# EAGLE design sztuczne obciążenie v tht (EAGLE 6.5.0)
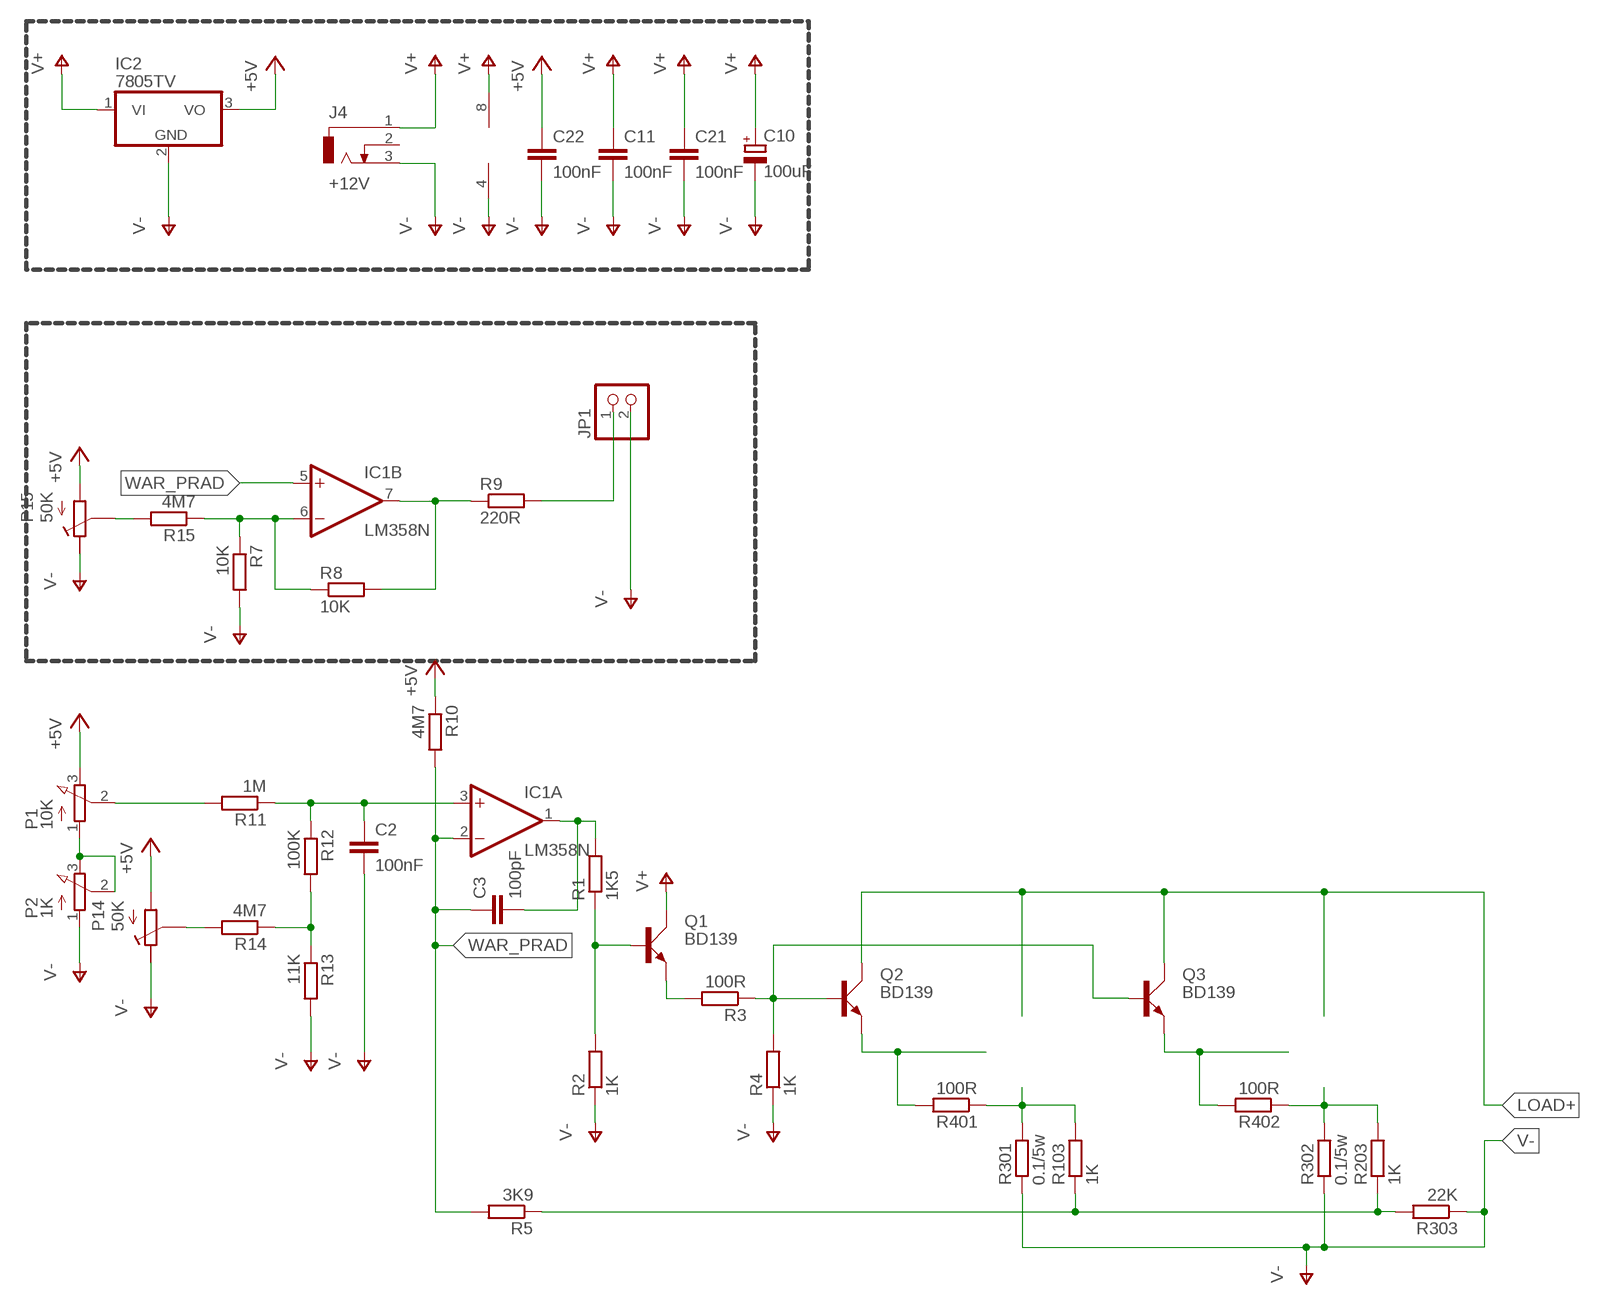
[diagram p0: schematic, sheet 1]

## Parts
C2  100nF  C-EU025-025X050  [C025-025X050]
C3  100pF  C-EU025-025X050  [C025-025X050]
C10  100uF  CPOL-EUE5-10.5  [E5-10,5]
C11  100nF  C-EU025-025X050  [C025-025X050]
C21  100nF  C-EU025-025X050  [C025-025X050]
C22  100nF  C-EU025-025X050  [C025-025X050]
IC1  LM358N  [DIL08]
IC2  7805TV  [TO220V]
J4  +12V  DCJ0202  [DCJ0202]
JP1  PINHD-1X2  [1X02]
P1  10K  3RP/1610N  [3RP/1610N]
P2  1K  3RP/1610N  [3RP/1610N]
P14  50K  POTENCJOMETR_RM-065  [RM065]
P15  50K  POTENCJOMETR_RM-065  [RM065]
Q1  BD139  [TO126AV]
Q2  BD139  [TO126AV]
Q3  BD139  [TO126AV]
R1  1K5  R-EU_0207/7  [0207/7]
R2  1K  R-EU_0207/7  [0207/7]
R3  100R  R-EU_0207/7  [0207/7]
R4  1K  R-EU_0207/7  [0207/7]
R5  3K9  R-EU_0207/7  [0207/7]
R7  10K  R-EU_0207/7  [0207/7]
R8  10K  R-EU_0207/7  [0207/7]
R9  220R  R-EU_0207/7  [0207/7]
R10  4M7  R-EU_0207/7  [0207/7]
R11  1M  R-EU_0207/7  [0207/7]
R12  100K  R-EU_0207/7  [0207/7]
R13  11K  R-EU_0207/7  [0207/7]
R14  4M7  R-EU_0207/7  [0207/7]
R15  4M7  R-EU_0207/7  [0207/7]
R103  1K  R-EU_0207/7  [0207/7]
R203  1K  R-EU_0207/7  [0207/7]
R301  0.1/5w  R-EU_0922/22  [0922/22]
R302  0.1/5w  R-EU_0922/22  [0922/22]
R303  22K  R-EU_0207/7  [0207/7]
R401  100R  R-EU_0207/7  [0207/7]
R402  100R  R-EU_0207/7  [0207/7]

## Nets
+5V: C22.1 IC2.3(VO) P1.3(E) P14.P$3(A) P15.P$3(A) R10.1
LOAD+: Q2.C Q3.C
N$2: R203.2 R302.2 R402.1
N$3: Q2.B Q3.B R3.1 R4.2
N$4: Q2.E R401.2
N$5: Q1.B R1.1 R2.2
N$7: JP1.1 R9.2
N$8: C3.2 IC1.1(A:OUT) R1.2
N$9: P1.2(S) R11.2
N$10: C2.1 IC1.3(A:+IN) R11.1 R12.1
N$11: R12.2 R13.1 R14.1
N$12: Q1.E R3.2
N$13: Q3.E R402.2
N$14: R5.1 R103.1 R203.1 R303.2
N$15: P14.P$1(S) R14.2
N$16: IC1.6(B:-IN) R7.1 R8.1 R15.1
N$17: P15.P$1(S) R15.2
N$18: R103.2 R301.2 R401.1
N$19: IC1.7(B:OUT) R8.2 R9.1
N$26: P1.1(A) P2.2(S) P2.3(E)
V+: C10.+ C11.1 C21.1 IC1.8(P:V+) IC2.1(VI) J4.1 Q1.C
V-: C2.2 C10.- C11.2 C21.2 C22.2 IC1.4(P:V-) IC2.2(GND) J4.3 JP1.2 P2.1(A) P14.P$2(E) P15.P$2(E) R2.1 R4.1 R7.2 R13.2 R301.1 R302.1 R303.1
WAR_PRAD: C3.1 IC1.2(A:-IN) IC1.5(B:+IN) R5.2 R10.2
Unconnected: J4.2

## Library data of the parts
C2 C3 C11 C21 C22 = rcl:C-EU: CAPACITOR, European symbol
C10 = rcl:CPOL-EU: POLARIZED CAPACITOR, European symbol
IC1 = linear:LM358: OP AMP also LM158; LM258; LM2904 Source: http://cache.national.com/ds/LM/LM158.pdf
IC2 = linear:78*: Positive VOLTAGE REGULATOR Source: http://cache.national.com/ds/LM/LM78L05.pdf http://www.fairchildsemi.com/ds/LM/LM7805.pdf
J4 = con-jack:DCJ0202: DC POWER JACK Source: DCJ0202.pdf; OC_FARNELL: unknown; OC_NEWARK: unknown
JP1 = pinhead:PINHD-1X2: PIN HEADER
P1 P2 = pot:3RP/1610N: 16mm Potentiometer one level Source: http://www.alphapotentiometers.net/html/16mm_pot_2.html
P14 P15 = POT_RM065:POTENCJOMETR_RM-065
Q1-Q3 = transistor-power:BD139: NPN TRANSISTOR
R1-R5 R7-R15 R103 R203 R301-R303 R401 R402 = resistor:R-EU_: RESISTOR, European symbol

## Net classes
1 pradowa: width 1.524 mm, clearance 0.508 mm
2 srednia: width 0.635 mm

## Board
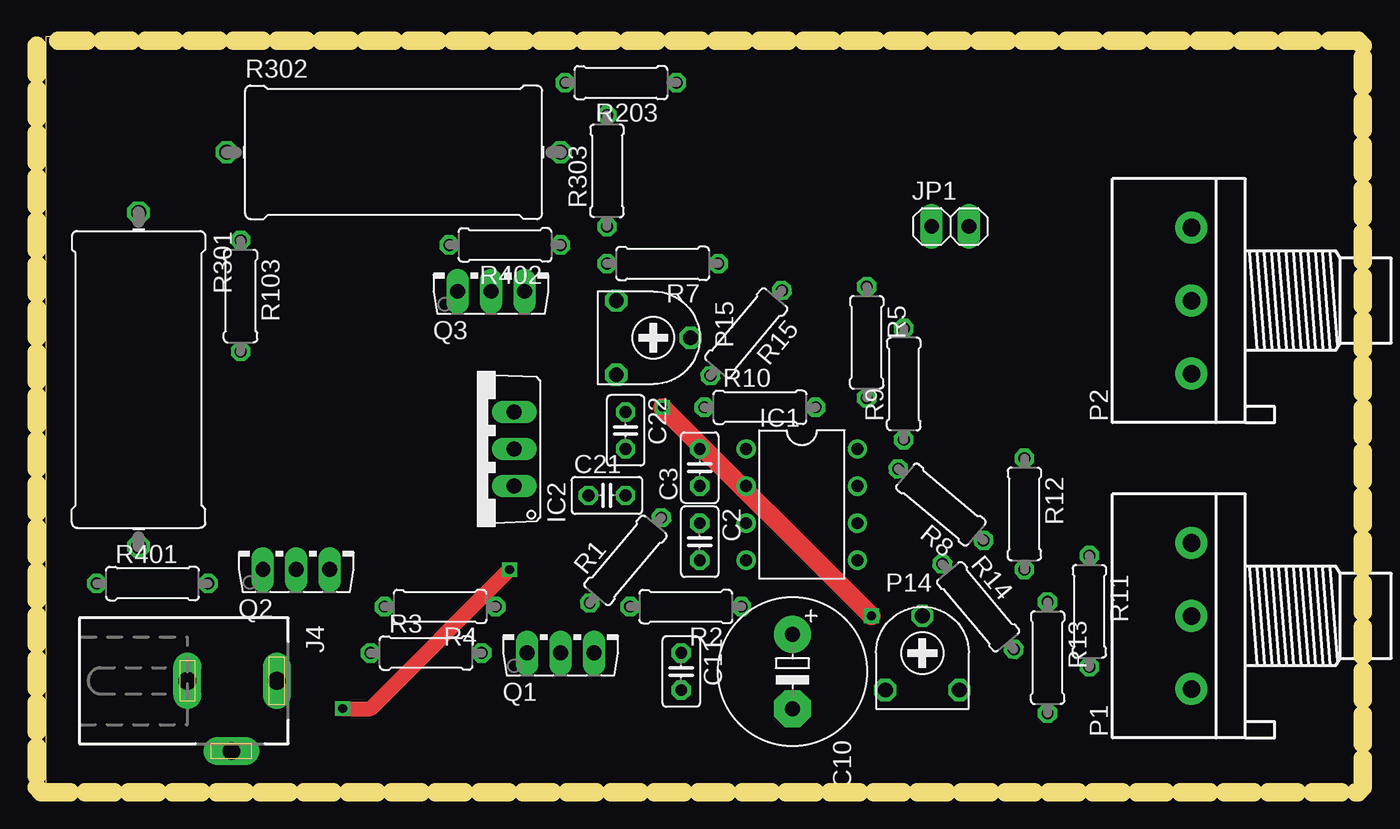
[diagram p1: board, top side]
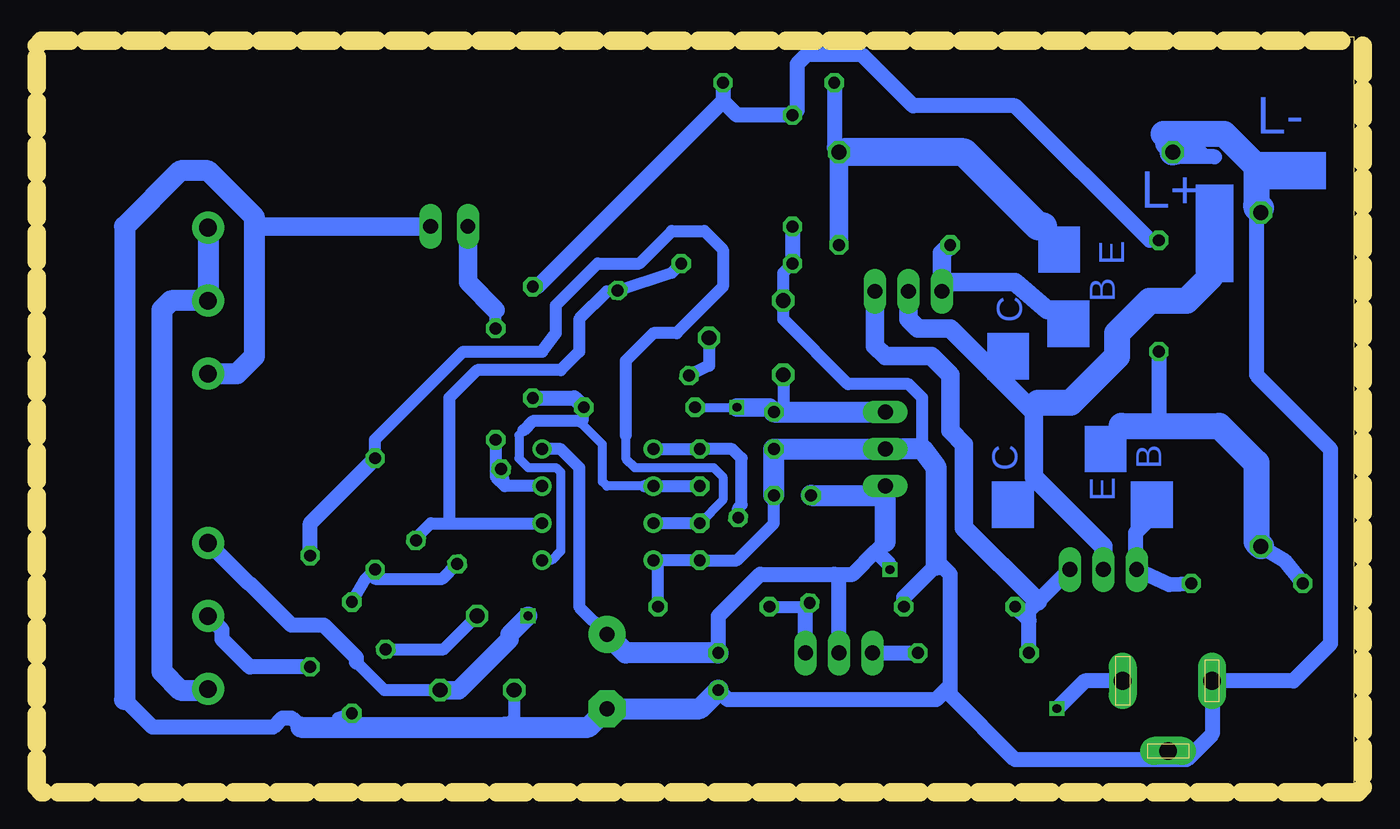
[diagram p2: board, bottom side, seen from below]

Size 90.81 x 51.74 mm. Coordinates in mm from the lower left corner, seen from the top.
Outline: 0.64,51.44 0.64,51.74 90.79,51.74 90.79,0.32 0.64,0 0.64,51.44
Outline: 0,51.12 0,0.32 0.32,0 90.49,0 90.81,0.32 90.81,51.12 90.49,51.44 0.64,51.44
Copper layers (1*16): Top 0.035mm / dielectric 1.5mm / Bottom 0.035mm
Design rules "default": minimum track width 10mil, minimum drill 24mil, track to track 8mil, track to pad 8mil, pad to pad 8mil, via to via 8mil, smd to smd 8mil, copper to edge 40mil, drill to drill 8mil, minimum pad ring 10mil, minimum via ring 8mil, stop-mask expansion 4mil, vias tented up to drill 0mil, thermal gap 10mil

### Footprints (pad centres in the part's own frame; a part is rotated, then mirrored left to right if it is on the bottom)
C025-025X050 = drill 0.813 octagon: 1 -1.27,0; 2 1.27,0
E5-10,5 = drill 1.016 pad 2.54: + -2.54,0 | drill 1.016 pad 2.54 octagon: - 2.54,0
DIL08 = drill 0.813 pad 1.27: 1 -3.81,-3.81; 2 -1.27,-3.81; 3 1.27,-3.81; 4 3.81,-3.81; 5 3.81,3.81; 6 1.27,3.81; 7 -1.27,3.81; 8 -3.81,3.81
TO220V = drill 1.016 long: 1 -2.54,-2.54; 2 0,-2.54; 3 2.54,-2.54
DCJ0202 = drill 1.2 pad 1.93 long: 1 0,3.105; 2 4.8,0; 3 0,-3.015
1X02 = drill 1.016 long: 1 -1.27,0; 2 1.27,0
3RP/1610N = drill 1.2 pad 2.184: 1 -5,0; 2 0,0; 3 5,0
RM065 = drill 1.016 octagon: P$1 0,2.54; P$2 -2.54,-2.54; P$3 2.54,-2.54
TO126AV = drill 1.016 long: B 2.286,-1.27; C 0,-1.27; E -2.286,-1.27
0207/7 = drill 0.813 octagon: 1 -3.81,0; 2 3.81,0
0922/22 = drill 1.016 octagon: 1 -11.43,0; 2 11.43,0

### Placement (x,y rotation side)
C2  45.4,17.14 270 top
C3  45.4,22.23 90 top
C10  51.75,8.26 270 top
C11  44.13,8.26 270 top
C21  39.05,20.32 0 top
C22  40.32,24.77 270 top
IC1  52.39,19.68 270 top
IC2  30.16,23.5 90 top
J4  13.33,7.62 270 top
JP1  62.55,38.73 0 top
P1  79.06,12.06 90 top
P2  79.06,33.66 90 top
P14  60.64,9.53 0 top
P15  42.23,31.11 270 top
Q1  35.88,10.79 0 top
Q2  17.78,16.51 0 top
Q3  31.12,35.56 0 top
R1  40.32,15.88 50 top
R2  44.45,12.7 180 top
R3  26.67,9.53 0 top
R4  27.62,12.7 180 top
R5  56.83,30.8 270 top
R7  42.86,36.2 180 top
R8  61.91,19.68 140 top
R9  59.37,27.94 90 top
R10  49.53,26.35 0 top
R11  72.07,12.38 270 top
R12  67.63,19.05 270 top
R13  69.22,9.21 270 top
R14  64.45,12.7 310 top
R15  48.58,31.43 230 top
R103  13.97,33.97 270 top
R203  40,48.58 180 top
R301  6.98,28.26 270 top
R302  24.45,43.81 0 top
R303  39.05,42.55 90 top
R401  7.94,14.29 0 top
R402  32.07,37.47 180 top

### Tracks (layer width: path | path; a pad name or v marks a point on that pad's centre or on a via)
+5V  (via drill 0.6)
  Top 1.27: v57.15,12.06 v42.86,26.35
  Bottom 0.61: R10.1 v42.86,26.35
  Bottom 0.813: P14.P$3 66.99,6.99 68.9,8.89 | P15.P$3 39.69,26.04
  Bottom 1.016: 68.9,8.89 68.9,9.21 71.12,11.43 73.34,11.43 76.2,14.29 76.28,14.29 P1.3
  Bottom 1.27: P14.P$3 61.91,6.99 58.42,10.48 58.42,10.79 v57.15,12.06 | v42.86,26.35 40.64,26.35 C22.1
  Bottom 1.422: C22.1 39.69,26.04 IC2.3
LOAD+
  Bottom 1.27: Q2.C 17.78,16.83 22.54,21.59 22.54,26.04 28.26,31.75 30.48,31.75 31.12,32.38 Q3.C
N$1
  Bottom 1.27: 21.59,33.02 23.81,34.92 28.58,34.92
N$2
  Bottom 1.016: R203.2 36.2,44.13 R302.2
  Bottom 1.27: R402.1 R302.2
N$3
  Bottom 1.016: R3.1 22.86,11.75 | 22.86,11.75 R4.2 | 22.86,11.75 22.86,12.45 22.26,13.05 Q2.B
  Bottom 1.27: Q3.B 33.4,30.54 32.7,29.84 29.53,29.84 28.26,28.57 28.26,24.77 27.31,23.81 27.31,18.1 22.26,13.05
N$4
  Bottom 1.016: Q2.E 13.27,14.22 R401.2
N$5
  Bottom 0.813: R2.2 38.13,12.7 R1.1
  Bottom 1.016: Q1.B 38.16,12.67 R1.1
N$6
  Bottom 1.016: 15.56,15.24 15.56,17.78 13.97,19.37
N$7
  Bottom 0.813: R9.2 59.37,33.02
  Bottom 1.27: JP1.1 61.28,34.92 59.37,33.02
N$8
  Bottom 0.813: IC1.1 C3.2 43.18,23.5 42.54,22.86 42.54,19.68 42.77,19.46 R1.2
N$9
  Bottom 1.016: R11.2 76.2,8.57 78.11,10.48 78.11,11.11 P1.2
N$10
  Bottom 0.61: 50.48,24.45 50.48,22.86 49.85,22.23 44.45,22.23 43.81,21.59 43.81,20 C2.1
  Bottom 0.813: C2.1 IC1.3 | R12.1 67.63,24.13 61.59,30.16 56.2,30.16 55.24,31.43 55.24,33.34 52.39,36.2 49.53,36.2 47.31,38.42 45.09,38.42 43.81,37.15 43.81,34.61 46.99,31.43 48.58,31.43 50.48,29.53 50.48,24.45
  Bottom 1.016: R11.1 72.07,18.41 R12.1
N$11
  Bottom 0.813: R13.1 68.26,14.61 R12.2 67.63,14.61 63.02,14.61 R14.1
N$12
  Bottom 1.016: Q1.E R3.2
N$13
  Bottom 1.27: Q3.E 28.83,36.89 R402.2
N$14
  Bottom 1.016: R103.1 14.61,37.78 23.81,46.99 30.8,46.99 34.29,50.48 38.1,50.48 38.73,49.85 38.73,46.67 R303.2 42.86,46.35 43.81,47.31 | R203.1 43.81,47.31 | R5.1 56.52,34.61 43.81,47.31
N$15
  Bottom 0.813: R14.2 62.93,9.78 P14.P$1
N$16
  Bottom 0.813: R8.1 64.83,17.4 63.82,18.41 62.55,18.41 | 62.55,18.41 IC1.6 | R7.1 47.31,35.56 R15.1 51.75,34.29 53.66,32.38 53.66,30.16 54.93,28.89 60.64,28.89 62.55,26.99 62.55,18.41
N$17
  Bottom 0.813: P15.P$1 44.77,29.21 R15.2
N$18
  Bottom 1.016: R301.2 5.4,15.88 R401.1 | R103.2 13.97,25.08
  Bottom 1.778: 16.51,25.08 13.97,25.08 9.84,25.08 7.3,22.54 7.3,17.14 R301.2
N$19
  Bottom 0.813: IC1.7 58.74,20.95 | 58.74,20.95 R8.2 | R9.1 59.37,21.59 58.74,20.95
N$20
  Bottom 1.93: 21.91,38.73 22.23,38.73 27.31,43.81 35.56,43.81
N$21
  Bottom 1.778: 22.23,26.67 20,26.67 16.83,29.84 16.83,31.43 14.61,33.66 12.06,33.66 10.48,35.24 10.48,40.64
N$26
  Bottom 1.422: P2.3 P2.2 81.6,33.66 82.23,33.02 82.23,8.26 80.96,6.99 79.14,6.99 P1.1
V+  (via drill 0.6)
  Top 1.016: v20.96,5.71 22.86,5.71 v32.38,15.24
  Bottom 0.813: IC1.8 54.93,23.5 53.66,22.23 53.66,12.7 C10.+
  Bottom 1.016: C11.1 44.13,12.06 41.27,14.92 36.2,14.92 | 36.2,14.92 34.92,14.92 33.34,16.51 | 33.34,16.51 32.7,17.14 | Q1.C 35.88,14.61 36.2,14.92 | J4.1 19.05,7.62 v20.96,5.71 | v32.38,15.24 32.38,15.56 33.34,16.51
  Bottom 1.422: C11.1 50.48,9.53 C10.+ | 32.7,17.14 32.7,20.32 | 32.7,20.32 IC2.1 | C21.1 32.7,20.32
V-
  Bottom 0.813: P14.P$2 58.1,5.08 58.74,4.45 | R13.2 70.17,5.08 69.53,4.45 | C21.2 40.32,18.41 42.86,15.88 C2.2 IC1.4 48.26,15.56 R2.1 | R7.2 39.69,35.56 P15.P$2 39.69,32.38 35.24,27.94 31.12,27.94 30.16,26.99 30.16,23.5
  Bottom 1.016: 84.77,6.35 82.87,4.45 74.61,4.45 73.98,5.08 73.34,5.08 72.71,4.45 | R4.1 31.43,13.34 29.21,15.56 29.05,15.72 28.26,14.92 28.26,7.3 | C11.2 43.5,6.35 29.21,6.35 28.26,7.3 | R303.1 R7.2 | 28.26,7.3 28.26,6.67 23.81,2.22 12.06,2.22 10.32,3.97 J4.3 4.76,7.62 2.22,10.16 2.22,23.5 7.3,28.57 7.3,40.01 | R301.1 6.98,40.01 6.98,40.32 | 10.16,43.5 12.7,43.5 R302.1 11.11,43.81
  Bottom 1.27: JP1.2 75.57,38.73 75.88,38.42
  Bottom 1.422: C11.2 45.4,5.71 C10.- 53.02,4.45 58.74,4.45 69.53,4.45 72.71,4.45 | 29.21,15.56 29.21,22.23 30.16,23.5 IC2.2 C22.2 C21.2 | P2.1 77.07,28.66 75.88,29.84 75.88,38.42 75.88,39.37 79.06,42.55 80.96,42.55 84.77,38.73 84.77,6.35
  Bottom 1.778: 13.65,45.09 12.06,45.09 | 12.06,45.09 9.53,45.09 7.3,42.86 7.3,40.32 | 7.3,40.32 6.98,40.01 | 7.3,40.01 7.3,40.32 | R302.1 13.02,44.13 13.33,44.45 12.7,44.45 12.06,45.09
WAR_PRAD
  Bottom 0.61: 57.47,24.77 57.78,24.45 57.78,22.86 57.15,22.23 55.24,22.23 54.93,21.91 54.93,16.51 55.56,15.88 IC1.5 | 49.21,20.95 51.75,20.95 52.07,21.27 52.07,23.81 53.5,25.24 | 53.5,25.24 53.66,25.4 | R10.2 53.34,25.4 53.5,25.24
  Bottom 0.813: C3.1 IC1.2 49.21,20.95 | 53.66,25.4 56.83,25.4 57.47,24.77
  Bottom 1.016: R5.2 53.98,26.99 R10.2
(copper drawn outside any net)
  shapes: Bottom area x10

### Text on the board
Bottom: L- | L+ | E | B | C | B | C | E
